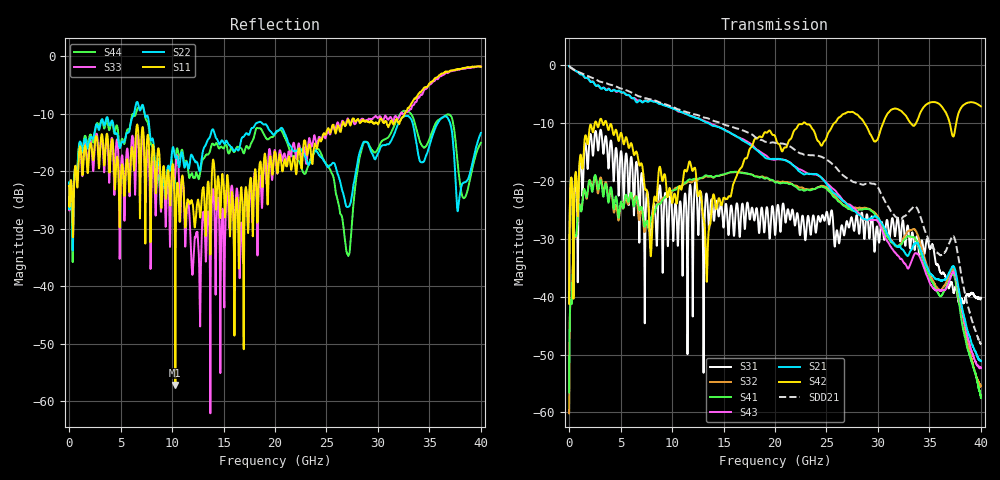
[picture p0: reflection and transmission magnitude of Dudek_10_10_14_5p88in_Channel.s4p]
! Created Thu Oct 09 16:28:59 2014
# hz S ma R 50
! 4 Port Network Data from SP1.SP block
! freq  magS11  angS11  magS12  angS12  magS13  angS13  magS14  angS14
!  magS21  angS21  magS22  angS22  magS23  angS23  magS24  angS24
!  magS31  angS31  magS32  angS32  magS33  angS33  magS34  angS34
!  magS41  angS41  magS42  angS42  magS43  angS43  magS44  angS44
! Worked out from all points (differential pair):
!   4001 points, 10 kHz to 40 GHz, reference 50 ohm
!   strongest paths, dB at 10 kHz, 10 GHz, 20 GHz, 30 GHz, 40 GHz:
!     S42: -41.2, -23.8, -12.2, -12.6, -7.1
!     S21: -0.2, -7.4, -16.2, -26.4, -51.2
!     S43: -0.2, -7.4, -16.3, -27.0, -52.2
!     S41: -56.6, -21.7, -20.2, -26.7, -57.5
!     S32: -60.2, -21.9, -20.2, -26.2, -55.3
!     S31: -41.1, -25.5, -29.2, -29.0, -40.2
!   taken as a pair (ports 1,3 in; 2,4 out), SDD21 dB: -0.1, -7.2, -13.4, -21.1, -48.2
!   lowest |S11| = -57.2 dB at 10.32 GHz (marker M1), VSWR 1.00, Z = 49.9 + j0.0992 ohm
!   |S11| at or under -10 dB: start of sweep to 32.59 GHz
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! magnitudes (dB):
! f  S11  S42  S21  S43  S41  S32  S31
! 10 kHz  -22.6  -41.2  -0.2  -0.2  -56.6  -60.2  -41.1
! 1.99 GHz  -15.8  -10.8  -2.7  -2.7  -19.9  -19.8  -12.6
! 10.32 GHz  -57.2  -22.6  -7.6  -7.6  -21.5  -21.2  -23.9
! 12.68 GHz  -27.1  -21.8  -9.3  -9.3  -19.5  -19.6  -23.7
! 27.09 GHz  -11.0  -8.1  -24.2  -24.0  -24.8  -24.5  -27.6
! 33.55 GHz  -7.3  -10.4  -30.9  -32.6  -29.8  -28.4  -31.9
! 40 GHz  -1.8  -7.1  -51.2  -52.2  -57.5  -55.3  -40.2
